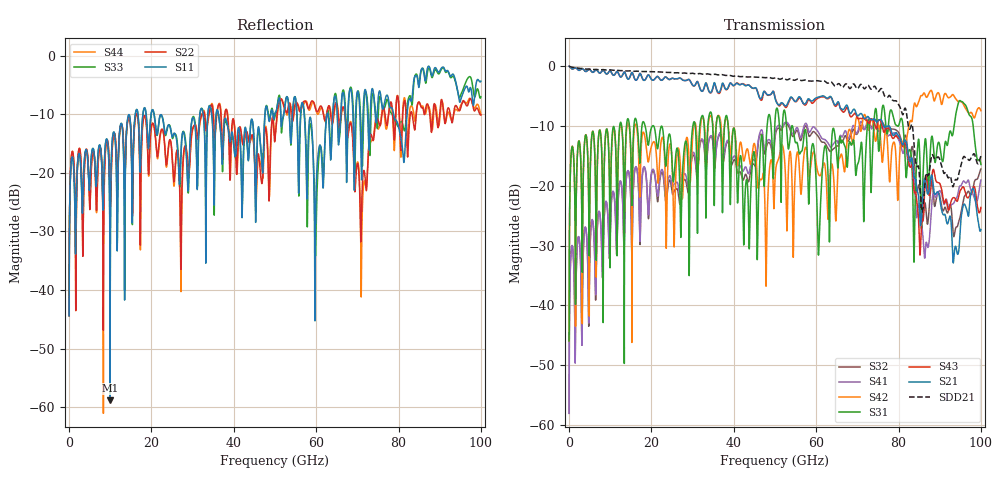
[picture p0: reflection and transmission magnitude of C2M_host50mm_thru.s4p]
# Hz S RI R 50
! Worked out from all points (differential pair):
!   10000 points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, 10 MHz to 100 GHz, reference 50 ohm
!   strongest paths, dB at 10 MHz, 25.01 GHz, 50.01 GHz, 75.01 GHz, 100 GHz:
!     S21: 0.0, -2.0, -5.4, -9.1, -27.3
!     S43: 0.0, -2.0, -5.2, -9.3, -23.6
!     S31: -45.9, -16.2, -9.2, -12.7, -16.5
!     S42: -45.9, -16.0, -18.9, -10.1, -7.5
!     S41: -58.0, -19.9, -11.5, -10.4, -19.1
!     S32: -58.0, -21.1, -12.0, -10.0, -17.2
!   taken as a pair (ports 1,3 in; 2,4 out), SDD21 dB: 0.0, -1.1, -2.0, -4.3, -15.0
!   lowest |S11| = -58.8 dB at 9.96 GHz (marker M1), VSWR 1.00, Z = 50.1 + j0.0101 ohm
!   |S11| at or under -10 dB: start of sweep to 16.08 GHz; 20.63 GHz to 31.74 GHz (11.12 GHz wide, 42.5 % of centre); 36.27 GHz to 47.56 GHz (11.28 GHz wide, 26.9 % of centre)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
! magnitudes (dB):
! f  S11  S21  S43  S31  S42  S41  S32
! 10 MHz  -44.4  0.0  0.0  -45.9  -45.9  -58.0  -58.0
! 750 MHz  -17.3  -0.5  -0.5  -13.4  -13.4  -30.0  -30.0
! 9.96 GHz  -58.8  -0.8  -0.8  -33.7  -23.3  -28.7  -28.9
! 59.93 GHz  -24.5  -5.3  -5.6  -18.3  -16.0  -10.5  -11.3
! 64.9 GHz  -7.8  -6.4  -6.7  -14.1  -24.6  -12.5  -13.4
! 71.06 GHz  -20.9  -8.0  -8.8  -12.9  -10.3  -9.3  -10.0
! 100 GHz  -4.4  -27.3  -23.6  -16.5  -7.5  -19.1  -17.2
